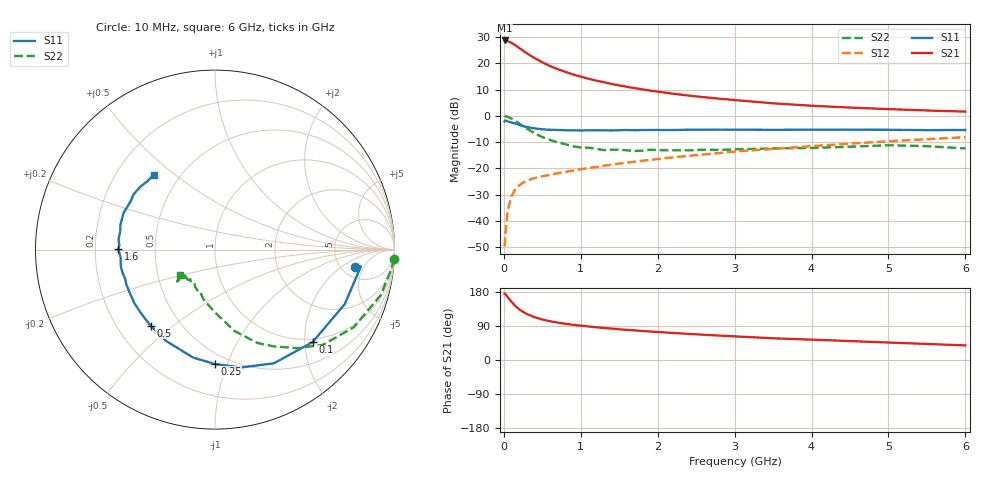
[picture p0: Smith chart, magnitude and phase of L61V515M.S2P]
!  INFINEON TECHNOLOGIES Small Signal Semiconductors
! BFR380L3 , Si-NPN RF-Transistor in TSLP-3-1
!  Vce=1.5 V,  Ic=15 mA
! Common Emitter S-Parameters:  07. March 2005
#  GHz  S  MA  R  50
! f  S11  S21  S12  S22
! GHz  Mag  Ang  Mag  Ang  Mag  Ang  Mag  Ang
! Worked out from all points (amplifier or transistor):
!   36 points, 10 MHz to 6 GHz, reference 50 ohm
!   highest |S21| = 28.7 dB at 10 MHz (marker M1)
!   |S21| within 3 dB of that: start of sweep to 206.4 MHz
!   unconditionally stable (mu >= 1): 1.978 GHz to 4.904 GHz
!   at 250 MHz: K = 0.31, MSG = 25.1 dB, |S12| = -25.4 dB
!   at 1.4 GHz: K = 0.92, MSG = 15.4 dB, |S12| = -18.6 dB
!   at 6 GHz: K = 0.98, MSG = 4.9 dB, |S12| = -8.1 dB
!   S11 on the Smith chart (normalised r, x): 10 MHz: 6.60, -3.35; 100 MHz: 0.92, -2.17; 250 MHz: 0.42, -0.90; 500 MHz: 0.34, -0.42; 1.6 GHz: 0.30, +0.00; 6 GHz: 0.36, +0.42
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0.01  0.7857 -7.1  27.34 175.3  0.0033 81.1  0.9994 -3.1
0.02  0.8181 -6.6  27.21 174.5  0.0055 84.5  0.9879 -6.3
0.05  0.784 -22.8  26.54 165.9  0.0158 80.3  0.9587 -15.2
0.1  0.7492 -43.5  24.54 153.3  0.0297 69.9  0.8861 -29.2
0.15  0.7136 -62.6  22.16 142.4  0.0401 62.3  0.8021 -41.4
0.2  0.6723 -77.6  19.65 133.7  0.0478 57.6  0.715 -50.2
0.25  0.6371 -90.2  17.47 127.0  0.0534 53.2  0.6303 -58.8
0.3  0.6139 -101.4  15.51 121.3  0.0581 50.9  0.572 -65.5
0.4  0.5774 -118.3  12.6 112.8  0.0655 48.4  0.465 -76.7
0.5  0.5555 -130.3  10.5 107.0  0.0709 47.9  0.3945 -83.5
0.6  0.5437 -139.7  8.912 102.3  0.0755 48.1  0.3487 -90.3
0.7  0.5393 -146.6  7.78 98.7  0.081 48.9  0.3126 -96.4
0.9  0.5308 -158.5  6.148 92.9  0.0907 51.1  0.2632 -106.7
1.1  0.5307 -165.8  5.11 88.4  0.1015 53.0  0.2479 -113.1
1.4  0.5269 -175.0  4.065 83.0  0.1176 55.3  0.2265 -120.9
1.6  0.5381 179.5  3.579 79.4  0.1286 56.4  0.2206 -128.9
2.2  0.5378 168.6  2.65 71.3  0.1623 58.8  0.2206 -133.3
2.8  0.5483 159.0  2.126 64.5  0.1962 60.3  0.2248 -139.9
3.5  0.5415 150.0  1.735 57.3  0.2352 59.5  0.24 -139.8
4.5  0.546 143.3  1.44 50.0  0.2961 59.0  0.2589 -140.0
5.5  0.5355 134.7  1.268 42.4  0.3597 56.0  0.2651 -140.6
6  0.5385 129.4  1.206 38.5  0.3932 54.1  0.2398 -143.3
